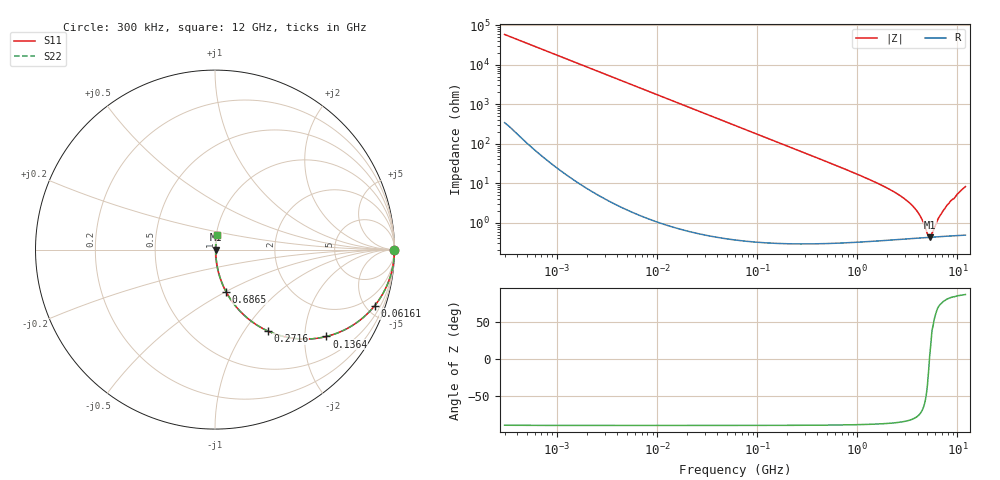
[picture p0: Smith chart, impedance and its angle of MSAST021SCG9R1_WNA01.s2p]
! MSAST021SCG9R1_WNA01  S-PARAMETER MODEL  ( General Type )
! Model Generated by TAIYO YUDEN Corporation (http://www.ty-top.com)
! Version 2.0
! TAIYO YUDEN Control No. 181101
! Copyright(c) 2015 TAIYO YUDEN CO.,LTD. All Rights Reserved.
! Product Description (link to TY-COMPAS)
! https://ds.yuden.co.jp/TYCOMPAS/or/detail?pn=MSAST021SCG9R1CWNA01&u=M
! Products Name : Multilayer Ceramic Capacitors
! Characteristics :
!  Capacitance : 9.1 pF , Rated Voltage : 25V , TCC : CG / C0G
!  Case Size : 0.25 x 0.125 / 0.0098 x 0.0049 [mm/inch] , Thickness : 0.125 / 0.0049 [mm/inch]
!  (Conditions: Temperature = 25 degC , DC Bias Current/Voltage = 0A / 0V)
! External Node Assignments :
!  1  o---| |---o  2
! GND o---------o GND
! Frequency Range : 0.3MHz  -  12000MHz  [ 401 STEP ]
# MHz S RI R 50
! Freq[MHz].  S11 Real  S11 Imag  S21 Real  S21 Imag  S12 Real  S12 Imag  S22 Real  S22 Imag
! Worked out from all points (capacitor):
!   401 points, 300 kHz to 12 GHz, reference 50 ohm
!   read as one part in series: C = 9.1 pF near 316.3 kHz
!   lowest |Z| = 428 mohm at 5.279 GHz (marker M1)
!   series resonance near 5.254 GHz, so ESL is about 100 pH
!   S11 on the Smith chart (normalised r, x): 300 kHz: open; 61.61 MHz: 1.01, -5.68; 136.4 MHz: 1.01, -2.56; 271.6 MHz: 1.01, -1.28; 686.5 MHz: 1.01, -0.50; 12 GHz: 1.01, +0.16
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0.3  1 -0.00172  1.3e-05 0.00172  1.3e-05 0.00172  1 -0.00172
1.769972  0.9999 -0.0101  0.000111 0.0101  0.000111 0.0101  0.9999 -0.0101
10.44266  0.9964 -0.0595  0.00359 0.0595  0.00359 0.0595  0.9964 -0.0595
26.39317  0.9776 -0.1475  0.0224 0.1475  0.0224 0.1475  0.9776 -0.1475
60  0.8944 -0.3067  0.1056 0.3067  0.1056 0.3067  0.8944 -0.3067
61.61074  0.8893 -0.3132  0.1107 0.3132  0.1107 0.3132  0.8893 -0.3132
91.67136  0.784 -0.4107  0.216 0.4107  0.216 0.4107  0.784 -0.4107
136.3989  0.6212 -0.4839  0.3788 0.4839  0.3788 0.4839  0.6212 -0.4839
271.6094  0.2929 -0.4528  0.7071 0.4528  0.7071 0.4528  0.2929 -0.4528
353.9943  0.1962 -0.3942  0.8038 0.3942  0.8038 0.3942  0.1962 -0.3942
686.4755  0.0615 -0.2343  0.9385 0.2343  0.9385 0.2343  0.0615 -0.2343
2088.533  0.00849 -0.0696  0.9915 0.0696  0.9915 0.0696  0.00849 -0.0696
2870.14  0.00562 -0.0423  0.9944 0.0423  0.9944 0.0423  0.00562 -0.0423
3642.919  0.0046 -0.0246  0.9954 0.0246  0.9954 0.0246  0.0046 -0.0246
4270.516  0.00429 -0.0137  0.9957 0.0137  0.9957 0.0137  0.00429 -0.0137
5006.236  0.00423 -0.0031  0.9958 0.0031  0.9958 0.0031  0.00423 -0.0031
5278.635  0.00426 0.000287  0.9957 -0.000287  0.9957 -0.000287  0.00426 0.000287
5565.855  0.00431 0.00334  0.9957 -0.00334  0.9957 -0.00334  0.00431 0.00334
6524.734  0.00458 0.0128  0.9954 -0.0128  0.9954 -0.0128  0.00458 0.0128
7648.807  0.00512 0.0242  0.9949 -0.0242  0.9949 -0.0242  0.00512 0.0242
10511.28  0.00832 0.0595  0.9917 -0.0595  0.9917 -0.0595  0.00832 0.0595
12000  0.0114 0.0807  0.9886 -0.0807  0.9886 -0.0807  0.0114 0.0807
